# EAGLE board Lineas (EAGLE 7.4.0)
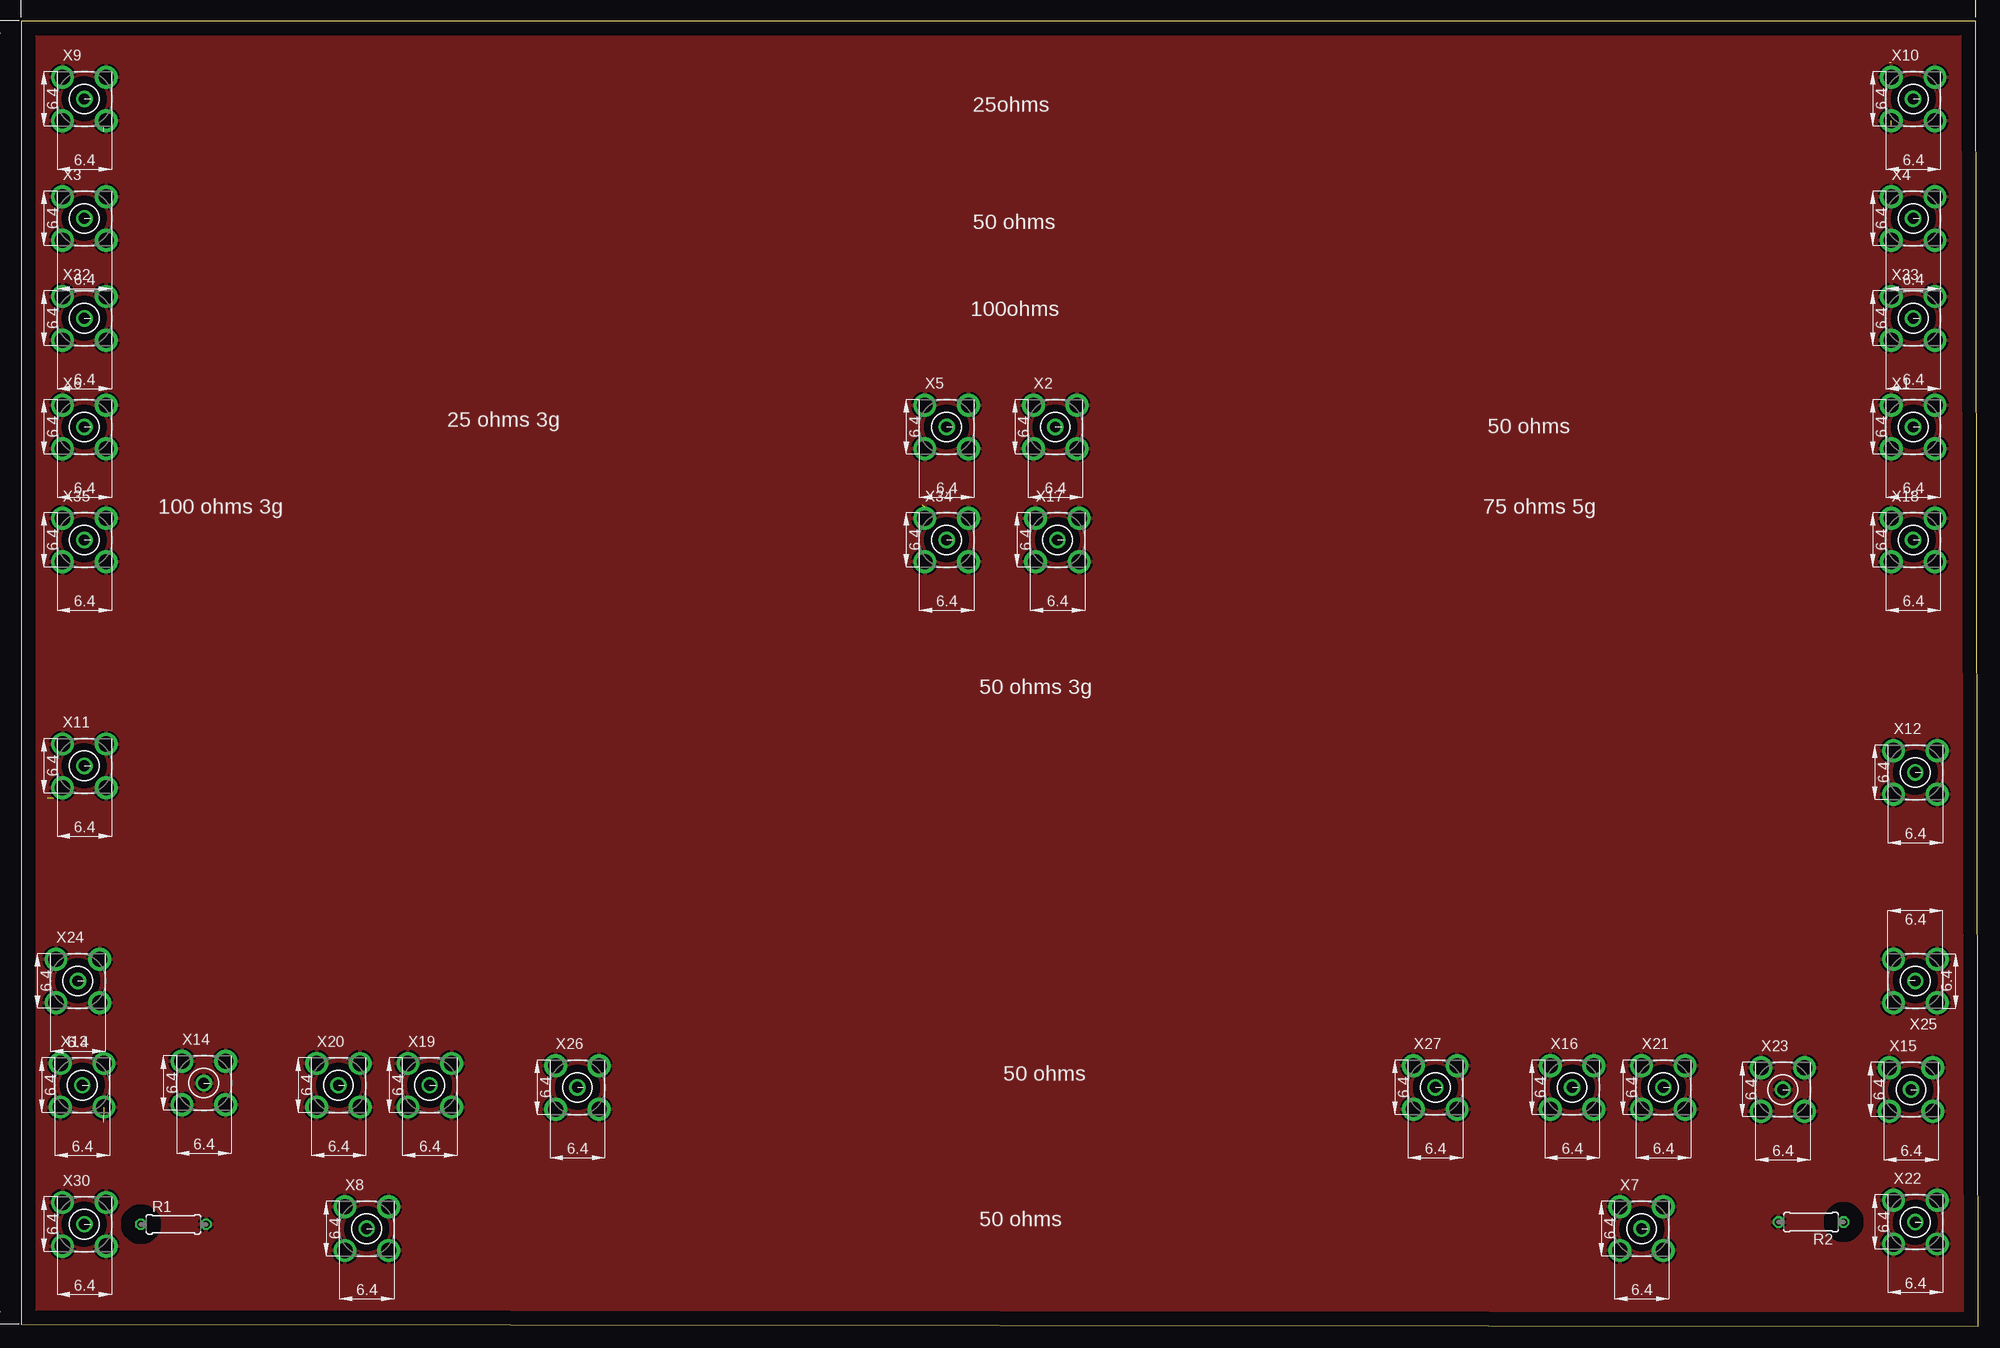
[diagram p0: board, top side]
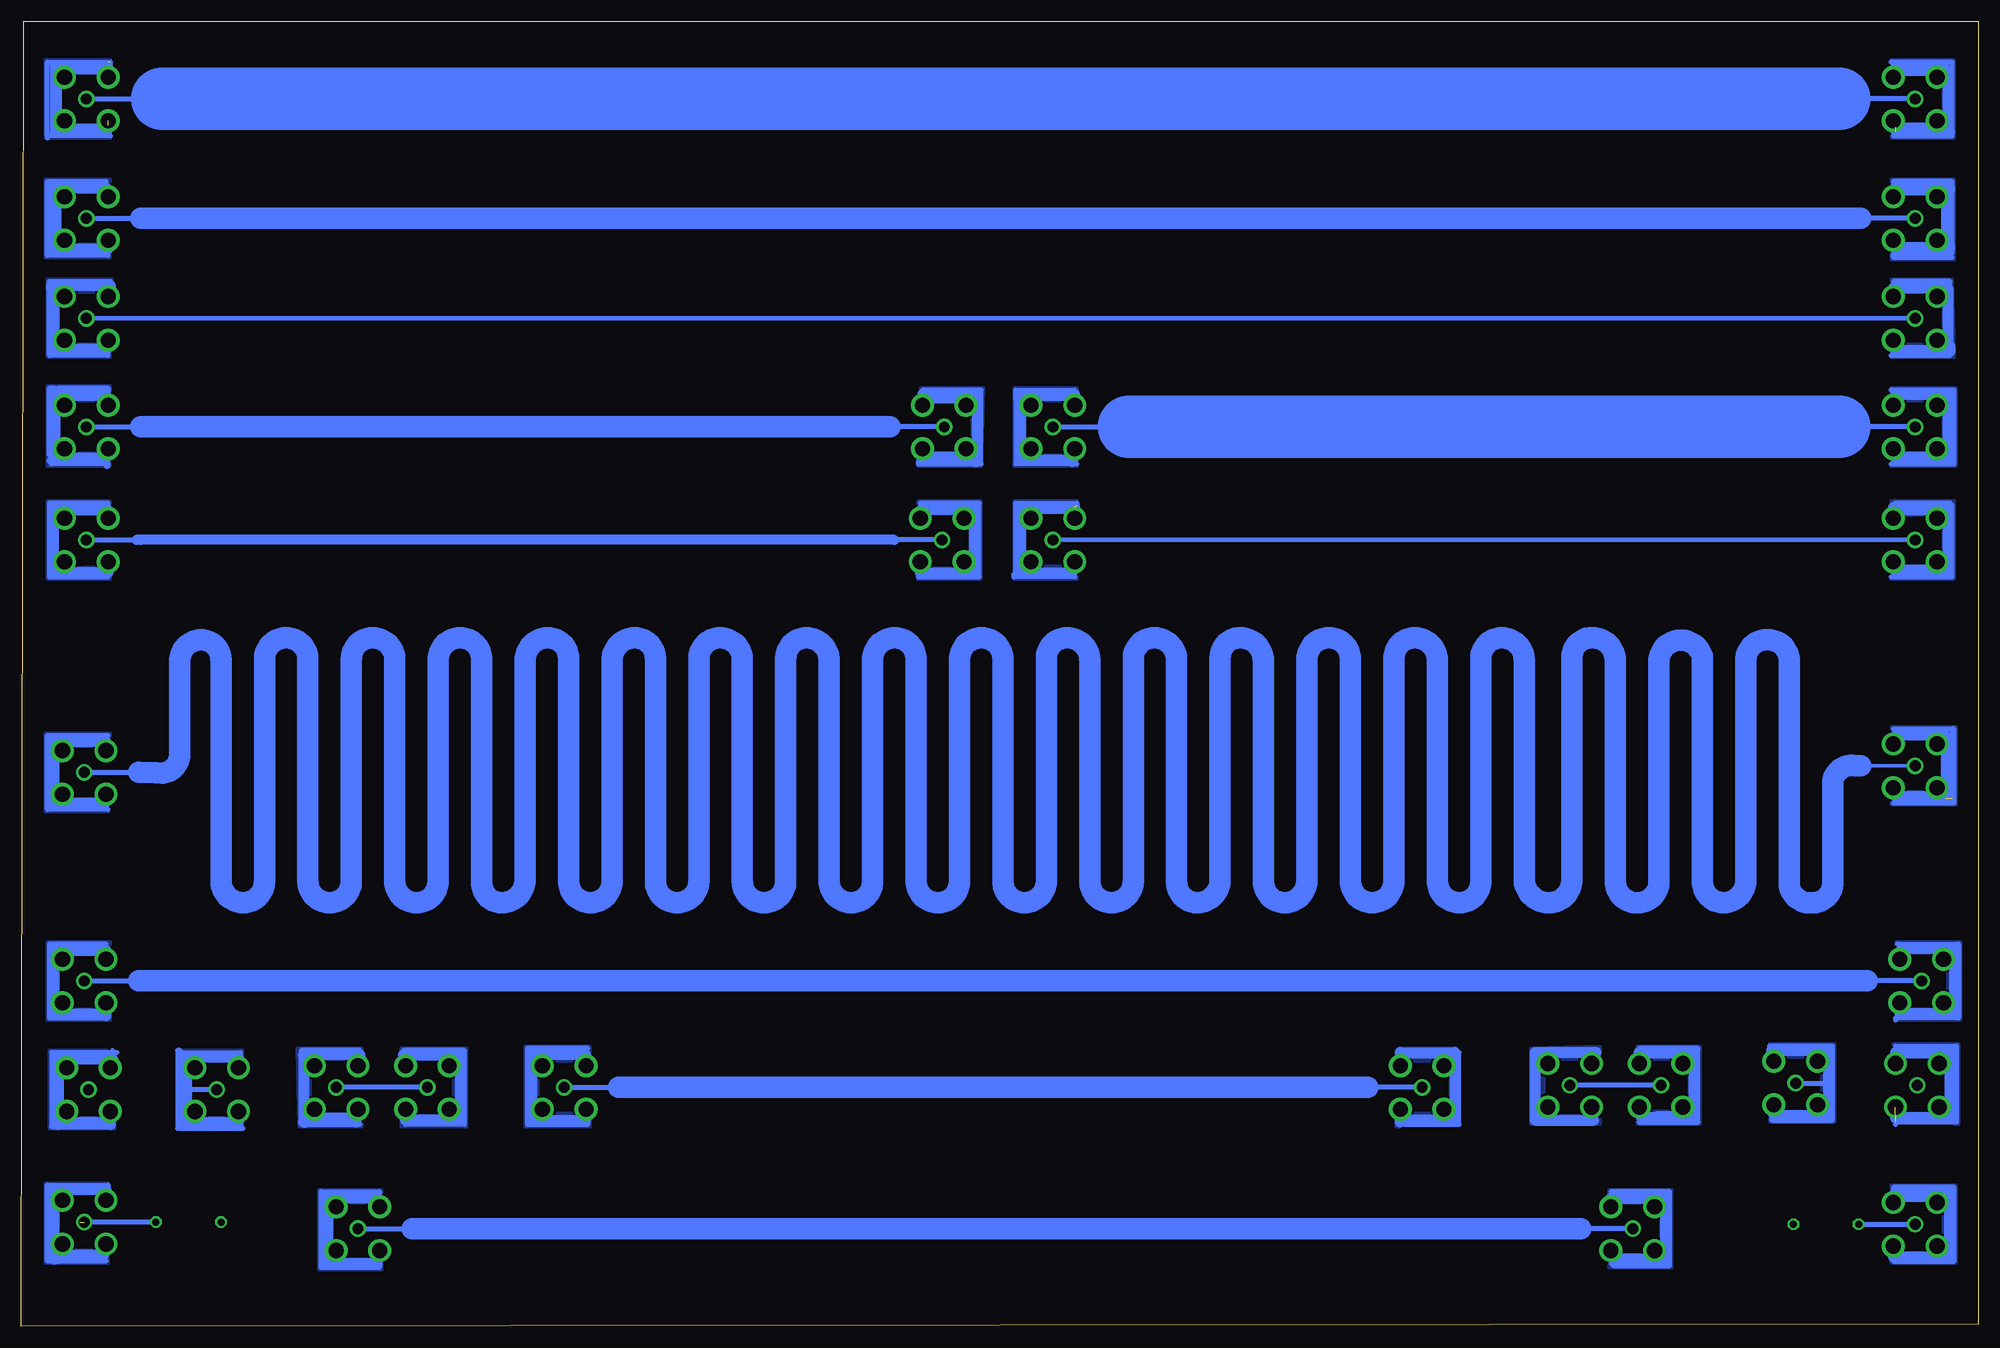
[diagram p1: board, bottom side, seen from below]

Size 228.83 x 152.58 mm. Coordinates in mm from the lower left corner, seen from the top.
Outline: 0,0.25 228.83,0 228.58,152.58 0,152.58 0,0.25
Copper layers (1*16): Top 0.035mm / dielectric 1.5mm / Bottom 0.035mm
Design rules "default": minimum track width 10mil, minimum drill 24mil, track to track 8mil, track to pad 8mil, pad to pad 8mil, via to via 8mil, smd to smd 8mil, copper to edge 40mil, drill to drill 8mil, minimum pad ring 10mil, minimum via ring 8mil, stop-mask expansion 4mil, vias tented up to drill 0mil, thermal gap 10mil

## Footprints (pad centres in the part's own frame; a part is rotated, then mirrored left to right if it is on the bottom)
0207/7 = drill 0.813 octagon: 1 -3.81,0; 2 3.81,0
BU-SMA-V = drill 1.27: 1 0,0 | drill 1.778: 2 -2.55,2.55; 3 2.55,2.55; 4 2.55,-2.55; 5 -2.55,-2.55

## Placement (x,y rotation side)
R1  50 ohms  [0207/7]  17.78,11.94 0 top
R2  75 ohms  [0207/7]  209.3,12.19 180 top
X1  BU-SMA-V  [BU-SMA-V]  221.23,105.16 0 top
X2  BU-SMA-V  [BU-SMA-V]  120.9,105.16 0 top
X3  BU-SMA-V  [BU-SMA-V]  7.37,129.54 0 top
X4  BU-SMA-V  [BU-SMA-V]  221.23,129.54 0 top
X5  BU-SMA-V  [BU-SMA-V]  108.2,105.16 0 top
X6  BU-SMA-V  [BU-SMA-V]  7.37,105.16 0 top
X7  BU-SMA-V  [BU-SMA-V]  189.48,11.43 0 top
X8  BU-SMA-V  [BU-SMA-V]  40.39,11.43 0 top
X9  BU-SMA-V  [BU-SMA-V]  7.37,143.51 0 top
X10  BU-SMA-V  [BU-SMA-V]  221.23,143.51 0 top
X11  BU-SMA-V  [BU-SMA-V]  7.37,65.53 0 top
X12  BU-SMA-V  [BU-SMA-V]  221.49,64.77 0 top
X13  BU-SMA-V  [BU-SMA-V]  7.11,28.19 0 top
X14  BU-SMA-V  [BU-SMA-V]  21.34,28.45 0 top
X15  BU-SMA-V  [BU-SMA-V]  220.98,27.69 0 top
X16  BU-SMA-V  [BU-SMA-V]  181.36,27.94 0 top
X17  BU-SMA-V  [BU-SMA-V]  121.16,91.95 0 top
X18  BU-SMA-V  [BU-SMA-V]  221.23,91.95 0 top
X19  BU-SMA-V  [BU-SMA-V]  47.75,28.19 0 top
X20  BU-SMA-V  [BU-SMA-V]  37.08,28.19 0 top
X21  BU-SMA-V  [BU-SMA-V]  192.02,27.94 0 top
X22  BU-SMA-V  [BU-SMA-V]  221.49,12.19 0 top
X23  BU-SMA-V  [BU-SMA-V]  205.99,27.69 0 top
X24  BU-SMA-V  [BU-SMA-V]  6.6,40.39 0 top
X25  BU-SMA-V  [BU-SMA-V]  221.49,40.39 180 top
X26  BU-SMA-V  [BU-SMA-V]  65.02,27.94 0 top
X27  BU-SMA-V  [BU-SMA-V]  165.35,27.94 0 top
X30  BU-SMA-V  [BU-SMA-V]  7.37,11.94 0 top
X32  BU-SMA-V  [BU-SMA-V]  7.37,117.86 0 top
X33  BU-SMA-V  [BU-SMA-V]  221.23,117.86 0 top
X34  BU-SMA-V  [BU-SMA-V]  108.2,91.95 0 top
X35  BU-SMA-V  [BU-SMA-V]  7.37,91.95 0 top

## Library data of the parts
R1 R2 = resistor
X1-X27 X30 X32-X35 = con-coax; OC_FARNELL: unknown; OC_NEWARK: unknown

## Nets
GND: R1.2 R2.2 X1.2 X1.3 X1.4 X1.5 X2.2 X2.3 X2.4 X2.5 X3.2 X3.3 X3.4 X3.5 X4.2 X4.3 X4.4 X4.5 X5.2 X5.3 X5.4 X5.5 X6.2 X6.3 X6.4 X6.5 X7.2 X7.3 X7.4 X7.5 X8.2 X8.3 X8.4 X8.5 X9.2 X9.3 X9.4 X9.5 X10.2 X10.3 X10.4 X10.5 X11.2 X11.3 X11.4 X11.5 X12.2 X12.3 X12.4 X12.5 X13.2 X13.3 X13.4 X13.5 X14.1 X14.2 X14.3 X14.4 X14.5 X15.2 X15.3 X15.4 X15.5 X16.2 X16.3 X16.4 X16.5 X17.2 X17.3 X17.4 X17.5 X18.2 X18.3 X18.4 X18.5 X19.2 X19.3 X19.4 X19.5 X20.2 X20.3 X20.4 X20.5 X21.2 X21.3 X21.4 X21.5 X22.2 X22.3 X22.4 X22.5 X23.1 X23.2 X23.3 X23.4 X23.5 X24.2 X24.3 X24.4 X24.5 X25.2 X25.3 X25.4 X25.5 X26.2 X26.3 X26.4 X26.5 X27.2 X27.3 X27.4 X27.5 X30.2 X30.3 X30.4 X30.5 X32.2 X32.3 X32.4 X32.5 X33.2 X33.3 X33.4 X33.5 X34.2 X34.3 X34.4 X34.5 X35.2 X35.3 X35.4 X35.5
N$1: X1.1 X2.1
N$2: X3.1 X4.1
N$3: X5.1 X6.1
N$4: X7.1 X8.1
N$5: X9.1 X10.1
N$6: X11.1 X12.1
N$7: X13.1
N$9: X17.1 X18.1
N$10: X15.1
N$17: R1.1 X30.1
N$18: X32.1 X33.1
N$19: X34.1 X35.1
N$41: R2.1 X22.1
N$47: X24.1 X25.1
N$50: X26.1 X27.1
THRU_1: X19.1 X20.1
THRU_2: X16.1 X21.1

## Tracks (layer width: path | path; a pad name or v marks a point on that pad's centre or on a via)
GND  (6 unrouted)
  Bottom 0.406: X23.1 206.25,27.69 | 218.95,146.56 225.3,146.56 | 225.3,146.56 225.3,146.81 | 225.3,147.07 225.3,147.32 225.04,147.32 | 225.04,147.32 223.01,147.32 | 219.2,147.32 218.69,147.32 218.69,147.07 225.3,147.07 | 225.3,147.07 225.3,146.81 | 225.3,146.81 218.69,146.81 218.69,147.83 219.2,147.83 219.2,147.32 | 219.2,147.32 223.01,147.32 | 223.01,147.32 223.01,147.57 224.28,147.57 | 224.54,147.57 224.28,147.57 | 224.28,147.57 224.28,140.46 | 224.28,140.21 224.28,139.45 224.54,139.45 | 224.79,139.45 224.54,139.45 | 224.54,139.45 224.54,146.3 224.79,146.3 224.79,139.19 225.04,139.19 225.04,147.32 | 225.3,146.56 225.3,139.45 218.44,139.45 218.44,139.7 224.03,139.7 224.03,139.95 218.69,139.95 218.69,140.21 224.28,140.21 | 224.28,140.21 224.28,140.46 | 224.28,140.46 218.69,140.46
  Bottom 0.61: 42.93,7.37 42.67,7.37 42.67,7.11 36.07,7.11 36.07,15.75 42.93,15.75 | 37.59,24.89 33.53,24.89 33.53,24.64 39.62,24.64 39.62,23.88 32.77,23.88 32.77,32.51 39.62,32.51 | 24.13,24.13 17.02,24.13 17.02,32.77 24.38,32.77 | X14.1 17.53,28.45 | 209.8,27.69 210.06,27.69 210.06,27.94 | 206.25,27.69 209.8,27.69 | 209.8,27.69 209.8,27.18 | 9.91,7.87 9.91,7.62 2.79,7.62 2.79,16.26 9.91,16.26 | 9.65,32.77 2.54,32.77 2.54,23.88 9.65,23.88 9.65,23.62 | 9.4,44.7 2.29,44.7 2.29,36.07 9.65,36.07 9.65,35.81 | 186.94,6.86 193.8,6.86 193.8,15.75 186.94,15.75 186.94,15.49 | 218.95,7.62 225.81,7.62 225.81,16.51 218.69,16.51 218.69,16.26 | 217.68,32 225.3,32 225.3,23.37 218.44,23.37 | 210.31,32.26 210.57,32.26 210.57,23.11 | 202.95,23.11 210.31,23.11 210.31,32 203.2,32 | 189.23,32.26 196.09,32.26 196.09,23.62 189.23,23.62 | 177.04,32 177.04,23.62 183.9,23.62 | 177.04,32.26 184.15,32.26 | 162.56,32.51 169.67,32.51 169.67,23.62 162.56,23.62 | 218.95,44.7 225.55,44.7 225.55,36.07 219.2,36.07 | 9.91,61.21 2.79,61.21 2.79,69.85 3.05,69.85 | 9.91,69.85 3.05,69.85 | 3.05,69.85 3.05,61.72 | 10.16,87.63 3.05,87.63 3.05,96.01 3.3,96.01 3.3,96.27 9.65,96.27 | 10.16,100.84 2.79,100.84 2.79,109.47 10.16,109.47 | 10.16,113.54 3.3,113.54 3.3,122.17 9.91,122.17 | 3.05,124.97 9.91,124.97 9.91,125.48 3.05,125.48 3.05,133.86 9.91,133.86 9.91,133.6 | 9.91,139.19 3.05,139.19 3.05,147.83 10.16,147.83 | 105.41,108.46 112.52,108.46 | 112.52,108.46 112.52,100.84 105.41,100.84 | 112.52,108.46 112.52,109.47 105.66,109.47 | 123.95,101.09 123.95,100.84 116.59,100.84 116.59,109.47 123.44,109.47 | 105.66,87.63 112.78,87.63 112.78,87.88 112.52,87.88 112.52,96.27 105.41,96.27 105.41,96.01
  Bottom 0.61: 123.95,87.63 116.84,87.63 116.84,96.27 123.7,96.27 | 218.69,60.45 225.81,60.45 225.81,69.09 218.69,69.09 | 218.69,96.27 225.55,96.27 225.55,87.63 218.69,87.63 | 218.69,101.09 218.95,101.09 218.95,100.58 218.69,100.58 218.69,100.84 225.3,100.84 225.3,101.09 225.55,101.09 225.55,101.35 218.69,101.35 218.69,101.85 225.55,101.85 225.55,109.73 225.04,109.73 225.04,108.71 | 224.79,108.46 218.44,108.46 218.44,108.71 218.69,108.71 218.69,109.73 224.54,109.73 224.54,101.6 225.04,101.6 225.04,104.14 225.04,108.71 | 224.79,108.46 224.79,108.2 | 224.79,108.46 224.79,109.22 218.95,109.22 218.95,108.97 219.2,108.97 219.2,108.71 225.04,108.71 | 218.69,113.54 225.55,113.54 225.55,122.17 218.44,122.17 | 218.69,125.22 225.81,125.22 225.81,125.48 | 225.3,133.86 225.81,133.86 225.81,125.48 | 225.3,133.86 225.3,125.48 225.81,125.48 | 225.3,133.86 218.95,133.86 218.95,133.6 | 218.44,139.19 225.81,139.19 | 225.81,139.19 225.81,138.94 | 225.81,139.19 225.81,147.83 218.44,147.83 218.44,147.07
  Bottom 1.143: 9.65,69.09 3.81,69.09 3.81,61.98 | 3.81,61.72 3.81,61.98 | 3.81,61.98 9.65,61.98 | 3.81,132.59 3.81,125.73 | 3.81,125.48 3.81,125.73 | 3.81,125.73 3.3,126.24 3.3,125.98 4.32,125.98 | 4.32,125.98 9.4,125.98 9.65,126.24 4.57,126.24 4.32,125.98 | 9.65,133.35 3.56,133.35 3.3,133.1 3.3,132.84 | 9.91,132.84 3.81,132.84 | 3.3,139.7 9.65,139.7 | 9.65,140.21 3.81,140.21 3.56,140.46 3.56,146.81 4.06,147.32 9.65,147.32 9.65,146.81 4.06,146.81
  Bottom 1.27: 42.93,14.99 36.58,14.99 36.58,7.87 42.67,7.87 42.67,8.13 | 44.7,32 51.82,32 51.82,24.13 44.96,24.13 | 39.62,32 33.27,32 33.27,24.38 39.37,24.38 | 67.56,32 61.21,32 61.21,24.13 67.56,24.13 67.56,23.88 | 24.13,32.26 17.53,32.26 17.53,28.45 17.53,24.64 23.88,24.64 | 9.91,8.13 3.3,8.13 3.3,15.75 9.65,15.75 9.65,15.24 4.32,15.24 | 8.89,44.2 2.79,44.2 2.79,36.58 9.14,36.58 | 187.2,14.99 193.04,14.99 193.04,7.87 193.29,7.87 193.29,7.37 187.2,7.37 | 218.95,16 225.04,16 225.04,8.38 | 225.04,8.13 225.04,8.38 | 225.04,8.38 219.2,8.38 225.04,7.87 | 218.19,31.24 224.54,31.24 224.54,23.88 | 224.54,23.62 224.54,23.88 | 224.54,23.88 218.44,23.88 218.44,23.62 | 189.23,31.75 195.83,31.75 195.83,23.88 195.58,23.88 195.58,24.38 189.74,24.38 189.74,23.88 | 203.45,31.5 209.55,31.5 209.55,23.88 203.45,23.88 | 184.15,31.75 177.55,31.75 177.55,24.13 183.9,24.13 | 162.81,31.75 169.16,31.75 169.16,24.13 162.81,24.13 | 218.95,43.94 225.04,43.94 225.04,36.58 218.95,36.58 218.95,36.32 | 9.65,95.76 9.91,95.76 9.91,95.5 3.56,95.5 3.56,88.39 9.65,88.39 | 9.65,108.97 3.56,108.97 | 3.3,108.97 3.56,108.97 | 3.56,108.97 3.56,101.6 | 3.56,101.35 3.56,101.6 | 3.56,101.6 9.65,101.6 | 9.91,121.41 3.56,121.41 3.56,114.55 3.3,114.55 3.3,114.05 9.65,114.05 9.65,114.3 | 105.66,108.97 112.01,108.97 112.01,101.35 105.92,101.35 105.92,101.09 | 123.44,108.97 117.09,108.97 117.09,101.09 117.35,101.09 117.35,101.6 123.44,101.6 | 105.66,95.76 112.01,95.76 112.01,88.14 105.92,88.14 | 123.7,88.14 117.35,88.14 117.35,95.5 123.44,95.5 123.44,95.76 | 218.95,68.33 225.04,68.33 225.04,61.21 219.2,61.21 219.2,60.96 | 218.69,88.14 225.04,88.14 225.04,95.5 218.95,95.5 218.95,95.76
  Bottom 1.27: 218.44,121.67 225.3,121.67 225.3,121.41 225.04,121.41 225.04,114.3 218.95,114.3 218.95,114.05 | 218.95,133.1 224.79,133.1 | 225.04,133.1 224.79,133.1 | 224.79,133.1 224.79,125.98 218.69,125.98
  pour Top (isolate 1.676): 228.85,0 0,0.25 0,152.65 228.6,152.65
  pour Bottom: 186.69,7.87 192.53,7.87 192.53,14.48 186.69,14.48 186.69,16 194.06,16 194.06,6.6 186.69,6.6
  pour Bottom: 2.79,138.94 10.16,138.94 10.16,140.46 4.06,140.46 4.06,146.56 10.16,146.56 10.16,148.08 2.79,148.08
  pour Bottom: 2.79,124.71 10.16,124.71 10.16,126.49 4.06,126.49 4.06,132.59 10.16,132.59 10.16,134.11 2.79,134.11
  pour Bottom: 2.79,113.28 10.16,113.28 10.16,114.81 4.06,114.81 4.06,120.9 10.16,120.9 10.16,122.43 3.05,122.43
  pour Bottom: 2.54,100.58 10.16,100.58 10.16,102.11 4.06,102.11 4.06,108.2 10.16,108.2 10.16,109.73 2.54,109.73
  pour Bottom: 2.79,87.38 10.16,87.38 10.16,88.9 4.06,88.9 4.06,95 10.16,94.74 10.16,96.52 2.79,96.52
  pour Bottom: 105.41,101.85 111.51,101.85 111.51,108.2 105.41,108.2 105.41,109.73 112.78,109.73 112.78,100.58 105.41,100.58
  pour Bottom: 105.41,88.9 111.51,88.9 111.51,95 105.41,95 105.41,96.52 112.78,96.52 112.78,87.38 105.41,87.38
  pour Bottom: 116.59,100.58 123.95,100.58 123.7,102.11 117.6,102.11 117.6,108.2 123.7,108.2 123.7,109.73 116.33,109.73
  pour Bottom: 116.59,87.38 123.95,87.38 123.95,88.65 117.86,88.65 117.86,95 123.95,95 123.95,96.52 116.59,96.52
  pour Bottom: 218.44,88.9 224.79,88.65 224.54,95 218.44,95 218.44,96.52 225.81,96.52 225.81,87.38 218.44,87.38
  pour Bottom: 218.44,102.11 224.54,102.11 224.54,108.2 218.44,108.2 218.44,109.98 225.81,109.98 225.81,100.58 218.44,100.58
  pour Bottom: 218.44,114.81 224.54,114.81 224.54,120.9 218.19,120.9 218.19,122.43 225.81,122.43 225.81,113.28 218.44,113.28
  pour Bottom: 218.44,126.49 224.54,126.49 224.54,132.59 218.44,132.59 218.44,134.11 226.06,134.11 226.06,124.97 218.44,124.97
  pour Bottom: 218.44,140.46 224.54,140.46 224.54,146.56 218.44,146.56 218.44,148.08 226.06,148.08 226.06,138.94 218.44,138.94
  pour Bottom: 2.54,60.96 10.16,60.96 10.16,62.48 4.32,62.48 4.06,68.83 10.16,68.58 10.16,70.1 2.54,70.1
  pour Bottom: 9.65,43.69 3.56,43.69 3.56,37.08 9.65,37.08 9.65,35.81 2.03,35.81 2.03,44.96 9.65,44.96
  pour Bottom: 2.29,23.62 9.91,23.62 9.91,24.89 3.81,24.89 3.81,31.5 9.91,31.5 9.91,33.02 2.29,33.02
  pour Bottom: 2.54,7.37 10.16,7.37 10.16,8.64 4.06,8.64 4.06,14.73 10.16,14.73 10.16,16.51 2.54,16.51
  pour Bottom: 24.38,31.5 18.29,31.5 18.29,24.89 24.38,24.89 24.38,23.88 16.76,23.88 16.76,33.02 24.38,33.02
  pour Bottom: 32.51,23.62 39.88,23.62 39.88,25.15 33.78,25.15 33.78,31.24 39.88,31.24 39.88,32.77 32.51,32.77
  pour Bottom: 35.81,6.86 43.18,6.86 43.18,8.38 37.08,8.38 37.08,14.48 43.18,14.48 43.18,16 35.81,16
  pour Bottom: 44.2,24.64 50.8,24.64 50.8,31.24 44.2,31.24 44.2,32.77 52.32,32.51 52.32,23.62 44.2,23.62
  pour Bottom: 60.45,23.37 68.07,23.37 68.07,24.89 61.72,24.89 61.72,30.99 67.82,30.99 67.82,32.51 60.45,32.51
  pour Bottom: 162.31,24.89 168.4,24.89 168.4,30.99 162.31,30.99 162.31,32.77 169.93,32.77 169.93,23.37 162.31,23.37
  pour Bottom: 184.4,31.24 178.31,31.24 178.31,24.64 184.4,24.64 184.4,23.37 176.78,23.37 176.78,32.51 184.4,32.51
  pour Bottom: 188.98,24.64 195.07,24.64 195.07,31.24 188.98,31.24 188.98,32.51 196.6,32.51 196.34,23.37 188.98,23.37
  pour Bottom: 202.95,24.38 209.04,24.38 209.04,30.99 202.95,30.99 202.95,32.26 210.57,32.26 210.57,23.11 202.95,23.11
  pour Bottom: 217.93,24.38 224.03,24.38 224.03,30.99 217.93,30.99 217.93,32.26 225.55,32.26 225.55,23.11 217.93,23.11
  pour Bottom: 218.69,8.89 224.54,8.89 224.54,15.49 218.69,15.49 218.69,16.76 226.06,16.76 226.06,7.37 218.69,7.37
  pour Bottom: 218.44,37.08 224.54,37.08 224.54,43.69 218.44,43.69 218.44,44.96 225.81,44.96 225.81,35.81 218.44,35.81
  pour Bottom: 218.69,61.72 224.79,61.47 224.54,67.82 218.44,67.82 218.44,69.34 226.06,69.34 226.06,60.2 218.69,60.2
N$1
  Bottom 0.61: X1.1 213.11,105.16 | X2.1 130.81,105.16
  Bottom 2.54: 127.25,105.16 130.81,105.16 213.11,105.16 214.88,105.16
N$2
  Bottom 0.61: X4.1 214.38,129.54 | X3.1 15.24,129.54
  Bottom 2.54: 13.72,129.54 15.24,129.54 214.38,129.54 214.88,129.54
N$3
  Bottom 0.61: X5.1 98.81,105.16 | X6.1 16.51,105.16
  Bottom 7.325: 16.26,105.16 16.51,105.16 98.81,105.16 99.31,105.16
N$4
  Bottom 0.61: X8.1 49.02,11.43 | X7.1 180.85,11.43
  Bottom 1.93: 181.1,11.43 181.61,11.43
  Bottom 2.54: 46.48,11.43 49.02,11.43 180.85,11.43 181.61,11.43 183.13,11.43
N$5
  Bottom 0.61: X10.1 209.8,143.51 | X9.1 16.26,143.51
  Bottom 7.285: 16.26,143.51 209.8,143.51 212.34,143.51
N$6
  Bottom 0.406: X11.1 13.72,65.53 | 215.13,64.77 213.1,64.76
  Bottom 0.61: X12.1 215.14,64.77
  Bottom 2.54: 13.72,65.53 14.27,65.53 arc-90 17.02,63.8 17.02,51.69 arc90 19.43,49.53 arc90 22.1,51.69 22.1,78.08 arc-90 24.79,80.26 arc-90 27.18,77.88 27.18,52.13 arc90 29.77,49.53 arc90 32.26,52.01 32.26,78.4 arc-155 37.34,77.98 37.34,51.65 arc165 42.42,51.82 42.42,77.82 arc-90 45.12,80.52 45.23,80.52 arc-90 47.5,78.25 47.5,52.23 arc90 50.2,49.53 50.24,49.53 arc90 53.09,52.38 53.09,77.9 arc-90 55.7,80.52 arc-90 58.17,78.05 58.17,52.03 arc90 60.67,49.53 arc90 63.25,52.11 63.25,77.87 arc-90 65.9,80.52 arc-90 68.33,78.09 68.33,52.07 arc90 70.87,49.53 arc90 73.41,52.07 73.41,78.02 arc-90 75.91,80.52 75.95,80.52 arc-90 78.49,77.98 78.49,52.14 arc90 81.1,49.53 arc90 83.57,52 83.57,77.77 arc-90 86.31,80.52 arc-90 88.65,78.19 88.65,52.23 arc90 91.35,49.53 arc90 93.73,51.91 93.73,77.9 arc-90 96.34,80.52 arc-90 98.81,78.05 98.81,52.07 arc90 101.35,49.53 arc90 103.89,52.07 103.89,77.87 arc-90 106.54,80.52 106.56,80.52 arc-90 108.97,78.11 108.97,52.1 arc90 111.53,49.53 arc90 114.05,52.04 114.05,78 arc-90 116.56,80.52 arc-90 119.13,77.95 119.13,52.04 arc90 121.64,49.53 arc90 124.21,52.1 124.21,78 arc-90 126.72,80.52 arc-90 129.29,77.95 129.29,52.04 arc90 131.8,49.53 arc90 134.37,52.1 134.37,77.87 arc-90 137.02,80.52 arc-90 139.45,78.09 139.45,52.07 arc90 141.99,49.53 142.01,49.53 arc90 144.53,52.04 144.53,77.93 arc-90 147.12,80.52 arc-90 149.61,78.03 149.61,52.07 arc90 152.15,49.53 arc90 154.69,52.07 154.69,78.11 arc-90 157.1,80.52 arc-90 159.77,77.85 159.77,52.04 arc90 162.28,49.53 arc90 164.85,52.1 164.85,78.11 arc-90 167.26,80.52 arc-90 169.93,77.85 169.93,52.27 arc90 172.66,49.53 arc90 175.01,51.87 175.01,78 arc-90 177.52,80.52 arc-90 180.09,77.95 180.09,52.07 arc90 182.63,49.53 arc90 185.17,52.07 185.17,77.93 arc-90 187.76,80.52 arc-90 190.25,78.03 190.25,52.07 arc90 192.79,49.53 arc90 195.33,52.07 195.33,77.98 arc-90 197.87,80.52 arc-90 200.41,77.98 200.41,52.03 arc90 202.91,49.53 arc90 205.49,52.11 205.49,77.92 arc-90 207.83,80.26 arc-90 210.31,77.78 210.31,67.04 arc88 212.32,64.7 213.1,64.76 215.14,64.77
N$9
  Bottom 0.61: X18.1 214.88,91.95 | X17.1 126.75,91.95
  Bottom 1.143: 126.75,91.95 214.88,91.95 215.39,91.95
N$13
  Bottom 0.61: 218.19,32 218.19,32.26
N$17
  Bottom 0.61: R1.1 X30.1
N$18
  Bottom 0.501: X32.1 X33.1
N$19
  Bottom 0.501: X35.1 X34.1
N$20
  Bottom 0.406: 211.07,143.51 213.11,143
N$22
  Bottom 0.406: 14.99,142.75 15.49,141.99
N$28
  Bottom 0.406: 16,40.13 14.73,40.13 14.73,40.64
N$29
  Bottom 0.406: 13.21,105.92 14.48,107.19
N$31
  Bottom 0.406: 13.72,106.68 14.99,105.66
N$41  (1 unrouted)
  Bottom 0.406: R2.1 213.11,11.94
  Bottom 0.61: R2.1 222,12.19 222,11.94
N$47
  Bottom 0.61: X24.1 13.97,40.39 | X25.1 211.33,40.39
  Bottom 2.54: 12.95,40.39 13.97,40.39 211.33,40.39 215.14,40.39
N$50
  Bottom 0.61: X26.1 72.39,27.94 | X27.1 159,27.94 157.73,27.94
  Bottom 2.54: 71.37,27.94 72.39,27.94 157.73,27.94 159,27.94
N$55
  Bottom 1.27: 9.65,32 3.3,32 3.3,24.38 9.65,24.38 9.65,24.64
N$71
  Bottom 0.61: 67.06,23.62 60.71,23.62 60.71,32
N$86
  Bottom 0.61: 123.7,108.2 117.35,108.2
N$88
  Bottom 0.61: 105.66,95.25 111.25,95.25
THRU_1
  Bottom 0.61: X20.1 X19.1
THRU_2
  Bottom 0.61: X16.1 X21.1

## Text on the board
tPlace: 25ohms | 50 ohms | 100ohms | 25 ohms 3g | 50 ohms | 100 ohms 3g | 75 ohms 5g | 50 ohms 3g | 50 ohms | 50 ohms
